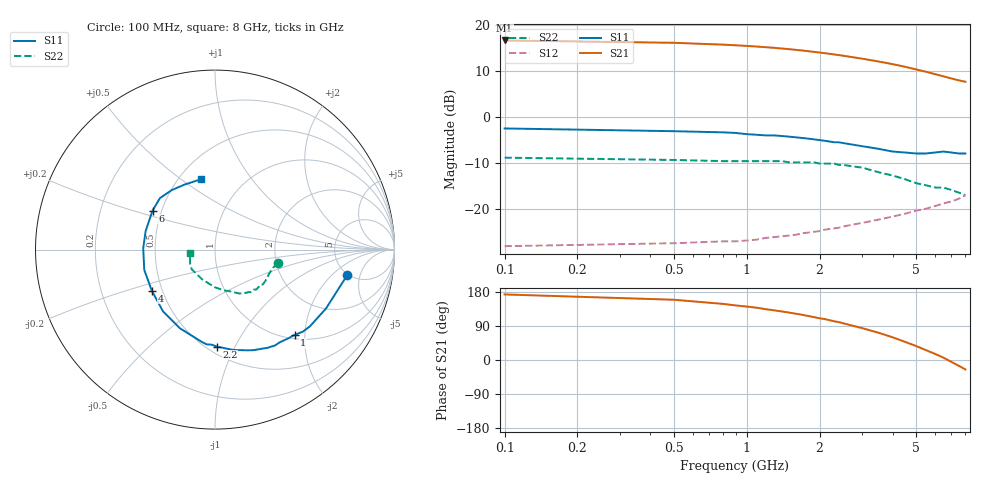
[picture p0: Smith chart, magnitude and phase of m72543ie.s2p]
!  MGA-72543 S PARAMETERS
!  Vd=3V  Id=40 mA Vc=0.3V  LAST UPDATED 01-27-99
# ghz s ma r 50
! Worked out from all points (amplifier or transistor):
!   31 points, 100 MHz to 8 GHz, reference 50 ohm
!   highest |S21| = 16.7 dB at 100 MHz (marker M1)
!   |S21| within 3 dB of that: start of sweep to 2.259 GHz
!   unconditionally stable (mu >= 1): start of sweep to end of sweep
!   at 1.1 GHz: K = 1.23, MAG = 18.2 dB, |S12| = -26.7 dB
!   at 2.1 GHz: K = 1.25, MAG = 16.2 dB, |S12| = -24.6 dB
!   at 8 GHz: K = 1.33, MAG = 8.9 dB, |S12| = -17.1 dB
!   lowest NFmin = 1.22 dB at 1 GHz
!   S11 on the Smith chart (normalised r, x): 100 MHz: 4.86, -3.18; 1 GHz: 1.08, -1.77; 2.2 GHz: 0.56, -0.85; 4 GHz: 0.44, -0.24; 6 GHz: 0.45, +0.23; 8 GHz: 0.64, +0.60
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0.1  0.75 -11.0  6.836 173.0  0.039 17.0  0.36 -12.0
0.5  0.7 -28.0  6.445 159.0  0.042 11.0  0.34 -17.0
0.8  0.68 -39.0  6.152 148.0  0.044 14.0  0.33 -24.0
0.9  0.67 -43.0  6.054 144.0  0.044 15.0  0.33 -26.0
1  0.65 -47.0  5.964 141.0  0.045 16.0  0.33 -28.0
1.1  0.64 -51.0  5.865 138.0  0.046 17.0  0.33 -30.0
1.2  0.63 -55.0  5.769 134.0  0.048 18.0  0.33 -32.0
1.4  0.62 -62.0  5.584 128.0  0.05 19.0  0.33 -36.0
1.6  0.6 -69.0  5.397 122.0  0.052 20.0  0.32 -40.0
1.9  0.57 -79.0  5.129 113.0  0.056 20.0  0.32 -44.0
2.2  0.54 -89.0  4.887 105.0  0.06 20.0  0.31 -49.0
2.5  0.52 -98.0  4.658 97.0  0.064 20.0  0.3 -53.0
3  0.48 -114.0  4.324 84.0  0.07 18.0  0.28 -61.0
3.5  0.45 -130.0  4.033 72.0  0.076 16.0  0.25 -69.0
4  0.42 -147.0  3.773 60.0  0.082 14.0  0.23 -79.0
4.5  0.41 -164.0  3.533 48.0  0.088 11.0  0.21 -90.0
5  0.4 179.0  3.306 37.0  0.095 7.0  0.19 -102.0
5.5  0.4 165.0  3.115 26.0  0.1 3.0  0.18 -114.0
6  0.41 148.0  2.932 16.0  0.107 0.0  0.17 -127.0
6.5  0.42 137.0  2.773 6.0  0.114 -5.0  0.17 -140.0
7  0.41 126.0  2.632 -5.0  0.12 -9.0  0.16 -150.0
8  0.4 101.0  2.422 -25.0  0.14 -18.0  0.14 -173.0
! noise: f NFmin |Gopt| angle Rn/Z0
0.8  1.29  0.4  36  0.27
1  1.22  0.35  41  0.27
1.8  1.49  0.26  61  0.23
2  1.52  0.24  68  0.22
2.2  1.53  0.24  75  0.22
2.4  1.55  0.23  81  0.21
3  1.59  0.22  100  0.18
4  1.64  0.2  142  0.14
5  1.71  0.23  -175  0.13
6  1.74  0.31  -133  0.15
